(* Logix 5000 AddOnInstructionDefinition export B256_ADJ; software revision 30.00 *)

ADD_ON_INSTRUCTION B256_ADJ   (* revision 1.0 20170916, vendor Kenneth A. Fischer *)
// if c >= m then subtract m
// Revision note:
// Rev1.0: 20170916 - Initial Release
VAR_IN_OUT
   Inp_C : DINT[22]; {required}
END_VAR
VAR
   i : INT;
   j : INT;
END_VAR

ROUTINE Logic   (* ladder *)
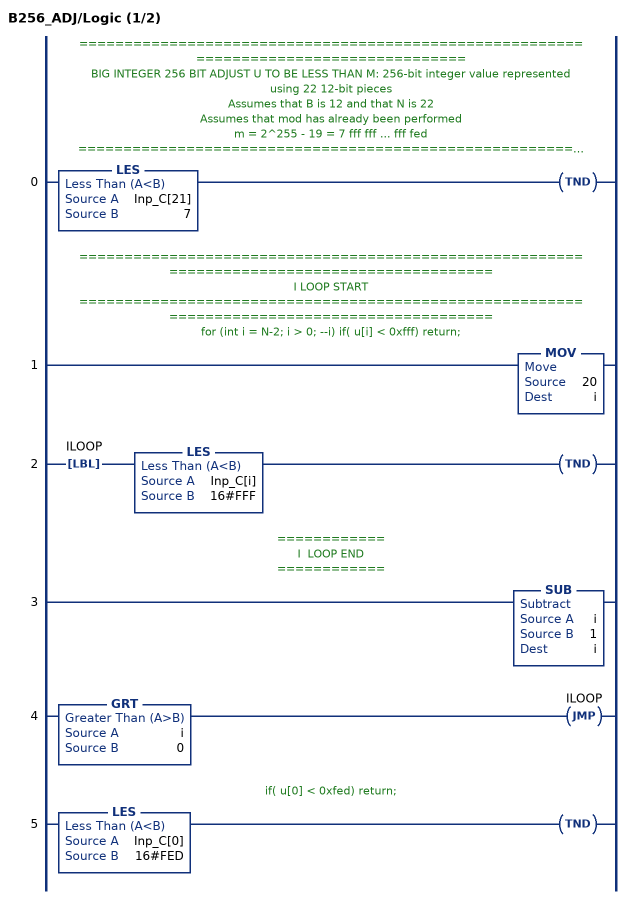
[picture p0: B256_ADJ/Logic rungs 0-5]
   // ======================================================================================
   // BIG INTEGER 256 BIT ADJUST U TO BE LESS THAN M: 256-bit integer value represented using 22 12-bit pieces
   // Assumes that B is 12 and that N is 22
   // Assumes that mod has already been performed
   // m = 2^255 - 19 = 7 fff fff ... fff fed
   // ======================================================================================
   // if (u[n-1] < 7) return;
   0: LES(Inp_C[21],7)TND();
   // ============================================================================================
   // I LOOP START
   // ============================================================================================
   // for (int i = N-2; i > 0; --i) if( u[i] < 0xfff) return;
   1: MOV(20,i);
   2: LBL(ILOOP)LES(Inp_C[i],16#FFF)TND();
   // ============
   // I  LOOP END
   // ============
   3: SUB(i,1,i);
   4: GRT(i,0)JMP(ILOOP);
   // if( u[0] < 0xfed) return;
   5: LES(Inp_C[0],16#FED)TND();
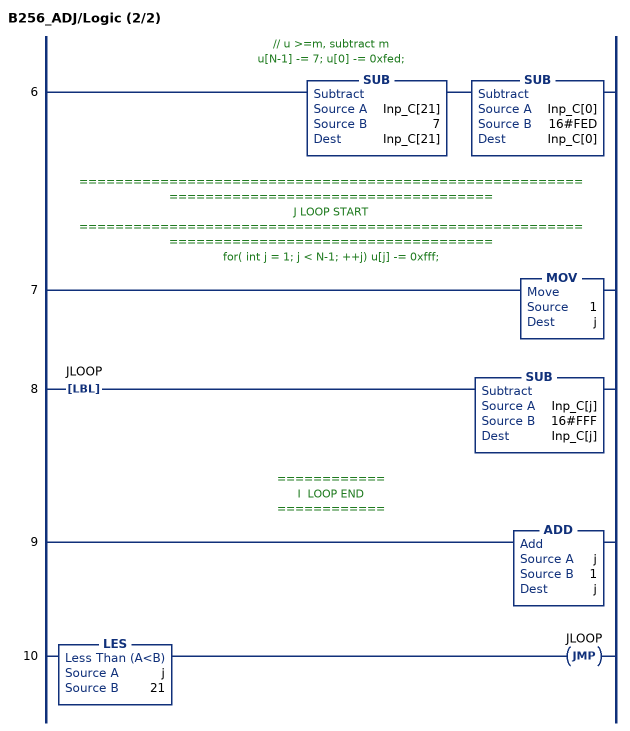
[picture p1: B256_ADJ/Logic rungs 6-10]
   // // u >=m, subtract m
   // u[N-1] -= 7; u[0] -= 0xfed;
   6: SUB(Inp_C[21],7,Inp_C[21])SUB(Inp_C[0],16#FED,Inp_C[0]);
   // ============================================================================================
   // J LOOP START
   // ============================================================================================
   // for( int j = 1; j < N-1; ++j) u[j] -= 0xfff;
   7: MOV(1,j);
   8: LBL(JLOOP)SUB(Inp_C[j],16#FFF,Inp_C[j]);
   // ============
   // I  LOOP END
   // ============
   9: ADD(j,1,j);
   10: LES(j,21)JMP(JLOOP);
END_ROUTINE
END_ADD_ON_INSTRUCTION
